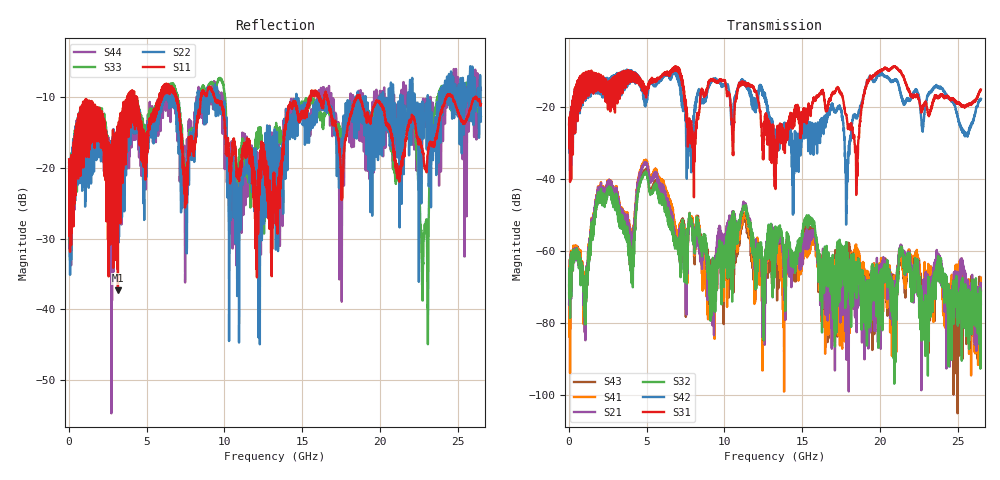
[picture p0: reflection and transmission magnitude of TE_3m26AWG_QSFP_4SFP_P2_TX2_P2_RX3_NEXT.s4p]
!Agilent Technologies,N5222A,MY51421691,A.10.00.00
!Agilent N5222A: A.10.00.00
!Date: Friday, January 30, 2015 12:35:50
!Correction: S11(Full 4 Port(1,2,3,4))
!S12(Full 4 Port(1,2,3,4))
!S13(Full 4 Port(1,2,3,4))
!S14(Full 4 Port(1,2,3,4))
!S21(Full 4 Port(1,2,3,4))
!S22(Full 4 Port(1,2,3,4))
!S23(Full 4 Port(1,2,3,4))
!S24(Full 4 Port(1,2,3,4))
!S31(Full 4 Port(1,2,3,4))
!S32(Full 4 Port(1,2,3,4))
!S33(Full 4 Port(1,2,3,4))
!S34(Full 4 Port(1,2,3,4))
!S41(Full 4 Port(1,2,3,4))
!S42(Full 4 Port(1,2,3,4))
!S43(Full 4 Port(1,2,3,4))
!S44(Full 4 Port(1,2,3,4))
!S4P File: Measurements: <S11,S12,S13,S14>,
!<S21,S22,S23,S24>,
!<S31,S32,S33,S34>,
!<S41,S42,S43,S44>:
# Hz S  dB  R 50.0
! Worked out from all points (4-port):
!   2650 points, 10 MHz to 26.5 GHz, reference 50 ohm
!   strongest paths, dB at 10 MHz, 6.63 GHz, 13.26 GHz, 19.88 GHz, 26.5 GHz:
!     S31: -24.8, -10.2, -30.3, -10.6, -15.3
!     S42: -25.1, -10.9, -28.9, -11.3, -17.9
!     S32: -69.6, -54.9, -63.5, -70.1, -71.4
!     S21: -71.7, -52.5, -64.5, -67.9, -74.7
!     S41: -66.4, -50.2, -61.3, -65.7, -67.4
!     S43: -74.7, -52.4, -62.1, -77.8, -71.0
!   lowest |S11| = -37.3 dB at 3.15 GHz (marker M1), VSWR 1.03, Z = 50.6 - j1.23 ohm
!   |S11| at or under -10 dB: start of sweep to 3.77 GHz; 9.336 GHz to 15.5 GHz (6.16 GHz wide, 49.6 % of centre); 18.72 GHz to 24.29 GHz (5.571 GHz wide, 25.9 % of centre)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
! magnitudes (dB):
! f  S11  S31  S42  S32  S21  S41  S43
! 10 MHz  -18.8  -24.8  -25.1  -69.6  -71.7  -66.4  -74.7
! 3.15 GHz  -37.3  -16.9  -14.4  -47.9  -45.6  -45.4  -47.4
! 17.87 GHz  -15.3  -23.3  -43.9  -57.6  -66.3  -79.2  -58.8
! 19.35 GHz  -12.8  -12.2  -11.7  -80.9  -74.3  -69.3  -74.1
! 22.74 GHz  -17.6  -20.8  -25.9  -84.1  -71.6  -76.5  -70.8
! 23.9 GHz  -12.5  -17.1  -14.4  -65.5  -62.4  -62.1  -64.6
! 26.5 GHz  -11.1  -15.3  -17.9  -71.4  -74.7  -67.4  -71.0
